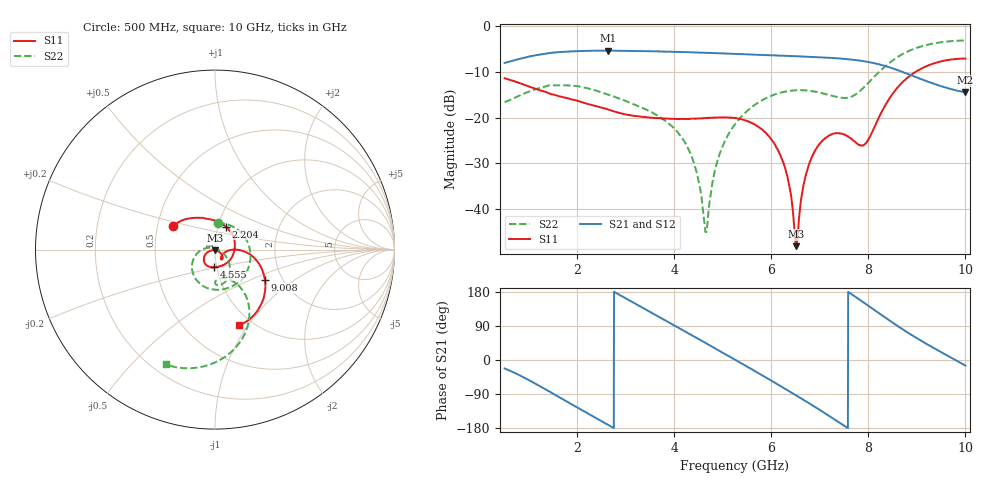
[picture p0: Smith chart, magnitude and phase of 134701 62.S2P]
!  2-Port S-parameters saved by WinCal
! VAR MeasName=S-Parameters (CALIBRATED_DATA) read from VNA (N5242A)
! VAR MeasDate=2013-7-3 16:41:19
! VAR NAME=134701 62
! VAR FILENAME=134701 62.S2P
! VAR DATE=2013-7-3 16:41:19
! VAR PHYS_PORTS=1,2
! VAR ObjTypeName=DATASET
! VAR IndexType=Frequency
# Hz S MA R 50
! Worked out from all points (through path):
!   1601 points, 500 MHz to 10 GHz, reference 50 ohm
!   highest |S21| = -5.37 dB at 2.632 GHz (marker M1); lowest = -14.5 dB at 10 GHz (marker M2)
!   group delay of S21, straight-line fit = 210 ps
!   lowest |S11| = -48.1 dB at 6.515 GHz (marker M3), VSWR 1.01, Z = 49.9 - j0.391 ohm
!   |S11| at or under -10 dB: start of sweep to 8.974 GHz
!   |S22| runs from -45.0 to -3.1 dB; largest |S21 - S12| = 0.0016
!   S11 on the Smith chart (normalised r, x): 500 MHz: 0.60, +0.17; 2.204 GHz: 1.09, +0.28; 4.555 GHz: 0.97, -0.19; 9.008 GHz: 1.63, -0.61; 10 GHz: 0.87, -0.91
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5e8  0.2685 151.0  0.3958 -22.4  0.3954 -22.3  0.1476 84.1
9.86875e8  0.2201 127.2  0.462 -52.2  0.462 -52.1  0.1913 4.9
1.438125e9  0.1823 107.8  0.5083 -84.2  0.5092 -84.2  0.2252 -50.6
2.085312e9  0.1482 73.5  0.5345 -131.6  0.5347 -131.6  0.2162 -104.5
2.204062e9  0.1413 65.4  0.5361 -140.2  0.5358 -140.3  0.2094 -112.1
2.631562e9  0.1231 31.1  0.5392 -171.1  0.5391 -171.1  0.1786 -133.9
3.670625e9  0.09868 -54.5  0.529 114.7  0.5283 114.7  0.1038 -167.3
4.2525e9  0.09653 -83.2  0.5183 73.0  0.5184 73.1  0.05002 170.8
4.555312e9  0.09813 -93.8  0.5126 51.2  0.5127 51.2  0.01379 140.1
4.662188e9  0.09926 -97.3  0.5099 43.6  0.51 43.6  0.005817 54.8
4.881875e9  0.1001 -105.0  0.5048 27.6  0.5056 27.6  0.03282 -15.9
5.25e9  0.09899 -119.2  0.4966 0.8  0.4968 0.8  0.08475 -36.0
6.122812e9  0.04533 -160.4  0.4771 -63.8  0.4767 -63.8  0.183 -69.6
6.336562e9  0.02186 -166.1  0.4722 -80.0  0.4723 -80.1  0.1943 -76.6
6.514688e9  0.003947 -97.1  0.4681 -93.7  0.4683 -93.8  0.199 -81.7
6.669062e9  0.01891 -28.3  0.4639 -105.7  0.4636 -105.8  0.1987 -85.4
6.835312e9  0.03705 -31.6  0.4602 -118.9  0.4604 -118.8  0.1949 -88.4
7.286562e9  0.06704 -51.6  0.4468 -155.2  0.4467 -155.3  0.1713 -87.4
7.915938e9  0.05061 -27.7  0.4128 150.5  0.4126 150.5  0.2155 -58.6
8.420625e9  0.1577 -2.9  0.3563 105.5  0.3558 105.4  0.3911 -60.7
9.008438e9  0.3245 -31.0  0.2734 56.9  0.2734 56.8  0.581 -81.5
1e10  0.4419 -72.3  0.1884 -14.8  0.1887 -14.8  0.6957 -113.3
